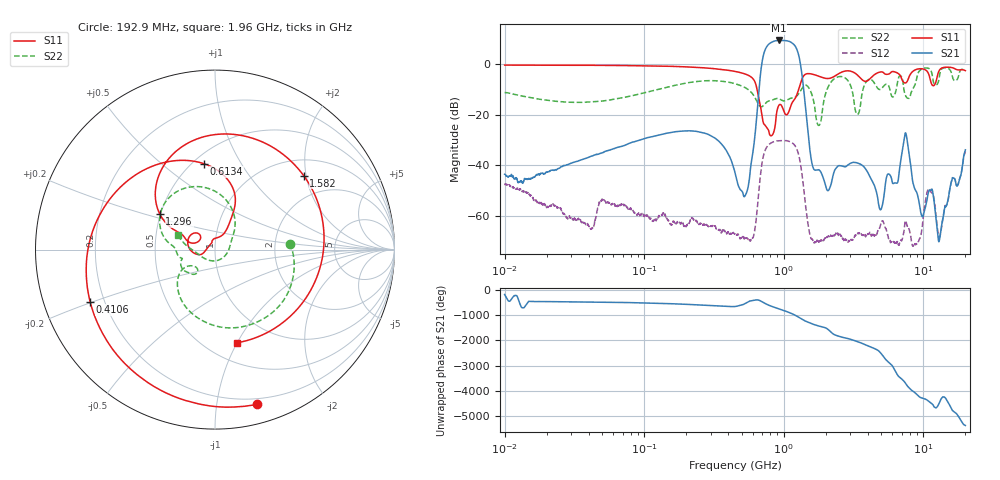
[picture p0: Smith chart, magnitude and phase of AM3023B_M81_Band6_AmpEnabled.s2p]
!Agilent Technologies,E8364B,MY43040894,A.07.50.67
!Agilent E8364B: A.07.50.67
!Date: Tuesday, October 27, 2020 10:44:14
!Correction: S11(Full 2 Port(1,2))
!S21(Full 2 Port(1,2))
!S12(Full 2 Port(1,2))
!S22(Full 2 Port(1,2))
!S2P File: Measurements: S11, S21, S12, S22:Log Frequency Sweep
# Hz S  dB  R 50
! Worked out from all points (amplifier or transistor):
!   3201 points, 10 MHz to 20 GHz, reference 50 ohm
!   highest |S21| = 9.5 dB at 922.9 MHz (marker M1)
!   |S21| within 3 dB of that: 745 MHz to 1.228 GHz (482.9 MHz wide, 49 % of centre)
!   unconditionally stable (mu >= 1): start of sweep to end of sweep
!   at 35.47 MHz: K = 4236.82, MAG = -26.9 dB, |S12| = -62.5 dB
!   at 447.2 MHz: K = 62997.63, MAG = -38.9 dB, |S12| = -67.2 dB
!   at 20 GHz: K = 234.32, MAG = -26.4 dB, |S12| = -34.4 dB
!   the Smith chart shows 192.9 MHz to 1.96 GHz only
!   S11 on the Smith chart (normalised r, x): 192.9 MHz: 0.15, -1.30; 410.6 MHz: 0.15, -0.20; 613.4 MHz: 0.57, +0.71; 1.296 GHz: 0.50, +0.23; 1.582 GHz: 1.38, +1.94; 1.96 GHz: 0.69, -1.00
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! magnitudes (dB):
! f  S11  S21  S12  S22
! 10 MHz  -0.3  -43.6  -47.6  -11.2
! 35.55 MHz  -0.4  -37.8  -62.5  -15.1
! 126.1 MHz  -0.7  -28.1  -60.5  -9.9
! 192.9 MHz  -1.0  -26.4  -64.1  -7.6
! 410.6 MHz  -2.5  -36.7  -67.2  -7.2
! 447.2 MHz  -2.8  -42.9  -67.2  -7.7
! 533.2 MHz  -3.9  -51.7  -69.3  -9.3
! 613.4 MHz  -6.3  -31.1  -67.0  -12.6
! 717.5 MHz  -23.5  4.0  -35.9  -16.2
! 922.9 MHz  -16.2  9.5  -30.3  -13.6
! 1.296 GHz  -8.7  2.2  -37.3  -11.1
! 1.582 GHz  -3.8  -38.5  -69.1  -11.6
! 1.59 GHz  -3.9  -39.1  -69.2  -12.0
! 1.96 GHz  -5.5  -46.6  -69.3  -13.1
! 3.482 GHz  -5.0  -39.4  -66.9  -18.4
! 4.948 GHz  -3.0  -57.6  -63.5  -9.8
! 5.639 GHz  -3.9  -43.4  -69.0  -8.5
! 7.499 GHz  -7.3  -27.4  -62.1  -12.7
! 9.692 GHz  -1.7  -59.7  -66.4  -2.0
! 11.07 GHz  -4.9  -49.8  -49.3  -1.8
! 13.01 GHz  -2.4  -69.8  -68.5  -4.8
! 20 GHz  -2.5  -33.9  -34.4  -2.3
